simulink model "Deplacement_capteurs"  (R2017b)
settings: Solver=ode15s  StartTime=0.0  StopTime=3  MaxStep=0.05  RelTol=1e-3  EnableMultiTasking=on
libraries: simulink x1

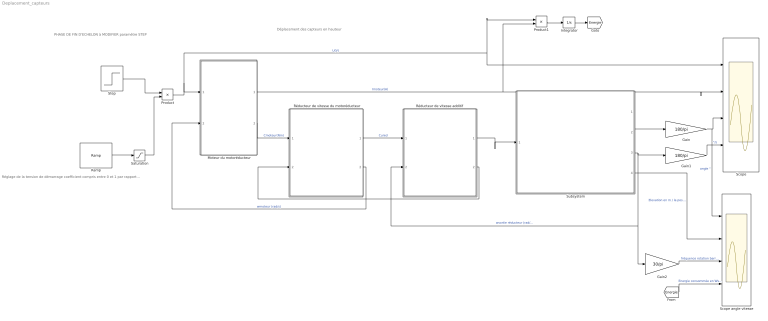
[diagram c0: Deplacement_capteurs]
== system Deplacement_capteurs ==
  note: Déplacement des capteurs en hauteur
  note: PHASE DE FIN D'ECHELON à MODIFIER paramètre STEP
  note: Réglage de la tension de démarrage coefficient compris entre 0 et 1 par rapport à ' initial input ex 0.25*(6V de l'autre bloc)= tension de démarrage à 1.5V
  Gain : Gain  Gain=180/pi
  Gain1 : Gain  Gain=180/pi
  Gain2 : Gain  Gain=30/pi
  Integrator : Integrator
  Moteur du motoréducteur : Subsystem  mask{R=1, K=0.08}
      mask prompts: R "Résistance interne"; K "K  en Nm/A ou V/(rad/s)"
  Product : Product
  Product1 : Product
  Ramp : simulink/Sources/Ramp  slope=1.5  start=0  X0=1
  "Réducteur de vitesse additif " : Subsystem  mask{KR=1/1, rend=1}
      mask prompts: KR "Rapport de réduction ws/we"; rend "rendement du réducteur"
  Réducteur de vitesse du motoréducteur : Subsystem  mask{KR=1/200, rend=0.65}
      mask prompts: KR "Rapport de réduction ws/we"; rend "rendement du réducteur"
  Saturation : Saturate  UpperLimit=1  LowerLimit=0
  Scope : Scope  NumInputPorts=4
  Scope angle vitesse : Scope  NumInputPorts=4
  Step : Step  Time=0.5  Before=1  After=0  SampleTime=0
  Subsystem : Subsystem  mask{m=1, long=0.37}
      mask prompts: m "masse en Kg soulevée"; long "longueur du bras"
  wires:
  Moteur du motoréducteur/2(cumot) -> Réducteur de vitesse du motoréducteur/1(Cmot)  "Cmoteur(Nm)"
  Réducteur de vitesse du motoréducteur/2(Wmoteur) -> Moteur du motoréducteur/2(rad/s)  "wmoteur (rad/s)"
  Product/1 -> Product1/1, Scope/1, Moteur du motoréducteur/1(U(v))  "U(V)"
  Gain/1 -> Scope angle vitesse/1, Scope/3  "angle °"
  Step/1 -> Product/1
  Saturation/1 -> Product/2
  Moteur du motoréducteur/1(I(A)) -> Product1/2, Scope/2  "Imoteur(A)"
  Gain1/1 -> Scope/4  "°/s"
  Subsystem/3(vitesse angulaire sortie bras rad/s) -> "Réducteur de vitesse additif "/2(W sort), Gain2/1, Gain1/1  "wsortie réducteur (rad/s)"
  Réducteur de vitesse du motoréducteur/1(Csortie) -> "Réducteur de vitesse additif "/1(Cmot)  "Cured"
  Subsystem/2(Angle rad) -> Gain/1
  Gain2/1 -> Scope angle vitesse/3  "fréquence rotation barre  trs/min"
  "Réducteur de vitesse additif "/2(Wmoteur) -> Réducteur de vitesse du motoréducteur/2(W sort)
  "Réducteur de vitesse additif "/1(Csortie) -> Subsystem/1(Cured)
  Subsystem/4(Elevation en m) -> Scope angle vitesse/2  "Elevation en m / la position 0"
  Product1/1 -> Integrator/1
  Integrator/1 -> [Energie]
  [Energie] -> Scope angle vitesse/4  "Energie consommée en Ws ou Joule"
  Ramp/1 -> Saturation/1

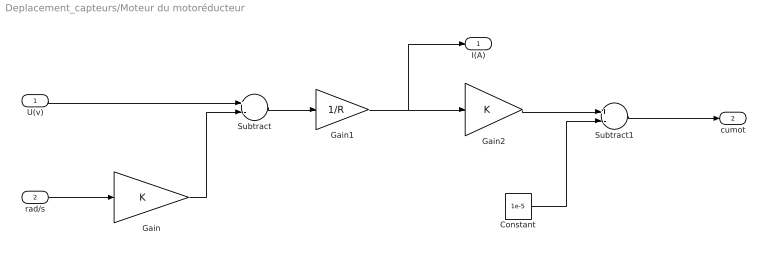
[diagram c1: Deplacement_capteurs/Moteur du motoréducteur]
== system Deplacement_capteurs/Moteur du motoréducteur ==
  U(v) : Inport
  rad/s : Inport  Port=2
  Constant : Constant  Value=1e-5
  Gain : Gain  Gain=K
  Gain1 : Gain  Gain=1/R
  Gain2 : Gain  Gain=K
  Subtract : Sum  Inputs=+-
  Subtract1 : Sum  Inputs=+-
  I(A) : Outport
  cumot : Outport  Port=2
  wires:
  U(v)/1 -> Subtract/1
  rad/s/1 -> Gain/1
  Gain/1 -> Subtract/2
  Subtract/1 -> Gain1/1
  Gain1/1 -> I(A)/1, Gain2/1
  Gain2/1 -> Subtract1/1
  Constant/1 -> Subtract1/2
  Subtract1/1 -> cumot/1

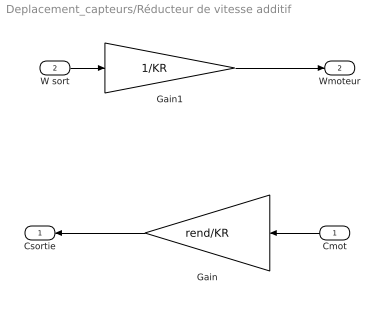
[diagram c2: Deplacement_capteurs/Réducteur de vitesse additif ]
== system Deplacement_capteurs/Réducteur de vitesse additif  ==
  Cmot : Inport
  W sort : Inport  Port=2
  Gain : Gain  Gain=rend/KR
  Gain1 : Gain  Gain=1/KR
  Csortie : Outport
  Wmoteur : Outport  Port=2
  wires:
  Cmot/1 -> Gain/1
  Gain/1 -> Csortie/1
  W sort/1 -> Gain1/1
  Gain1/1 -> Wmoteur/1

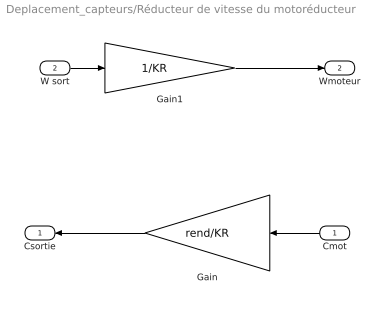
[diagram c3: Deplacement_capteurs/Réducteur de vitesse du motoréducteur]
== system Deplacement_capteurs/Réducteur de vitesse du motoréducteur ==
  Cmot : Inport
  W sort : Inport  Port=2
  Gain : Gain  Gain=rend/KR
  Gain1 : Gain  Gain=1/KR
  Csortie : Outport
  Wmoteur : Outport  Port=2
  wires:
  Cmot/1 -> Gain/1
  Gain/1 -> Csortie/1
  W sort/1 -> Gain1/1
  Gain1/1 -> Wmoteur/1

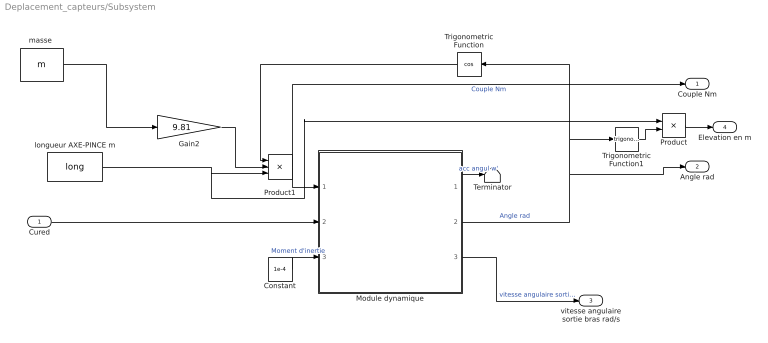
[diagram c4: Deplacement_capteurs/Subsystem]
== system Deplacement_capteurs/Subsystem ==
  Cured : Inport
  Constant : Constant  Value=1e-4
  Gain2 : Gain  Gain=9.81
  Module dynamique : Subsystem
  Product : Product
  Product1 : Product  Inputs=3
  Terminator : Terminator
  Trigonometric Function : Trigonometry  Operator=cos
  Trigonometric Function1 : Trigonometry
  longueur AXE-PINCE m : Constant  Value=long
  "masse " : Constant  Value=m
  Couple Nm : Outport
  Angle rad : Outport  Port=2
  vitesse angulaire sortie bras rad/s : Outport  Port=3
  Elevation en m : Outport  Port=4
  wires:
  Module dynamique/2(teta rad) -> Trigonometric Function/1, Trigonometric Function1/1, Angle rad/1  "Angle rad"
  Constant/1 -> Module dynamique/3(J)  "Moment d'inertie"
  Cured/1 -> Module dynamique/2(Cured)
  Module dynamique/3(W (rad/s)) -> vitesse angulaire sortie bras rad/s/1  "vitesse angulaire sortie bras rad/s"
  "masse "/1 -> Gain2/1
  Module dynamique/1(acc) -> Terminator/1  "acc angul w'"
  longueur AXE-PINCE m/1 -> Product/1, Product1/3
  Product1/1 -> Module dynamique/1(Cr), Couple Nm/1  "Couple Nm"
  Gain2/1 -> Product1/2
  Trigonometric Function/1 -> Product1/1
  Trigonometric Function1/1 -> Product/2
  Product/1 -> Elevation en m/1

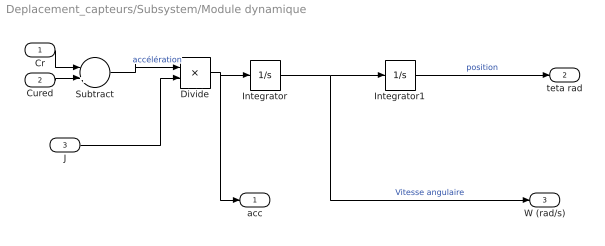
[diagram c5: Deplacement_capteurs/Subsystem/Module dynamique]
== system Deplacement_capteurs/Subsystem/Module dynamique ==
  Cr : Inport
  Cured : Inport  Port=2
  J : Inport  Port=3
  Divide : Product  Inputs=*/
  Integrator : Integrator
  Integrator1 : Integrator
  Subtract : Sum  Inputs=-+
  acc : Outport
  teta rad : Outport  Port=2
  W (rad/s) : Outport  Port=3
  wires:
  Integrator/1 -> Integrator1/1, W (rad/s)/1  "Vitesse angulaire"
  Cr/1 -> Subtract/1
  Integrator1/1 -> teta rad/1  "position"
  Cured/1 -> Subtract/2
  Subtract/1 -> Divide/1  "accélération"
  Divide/1 -> Integrator/1, acc/1
  J/1 -> Divide/2
